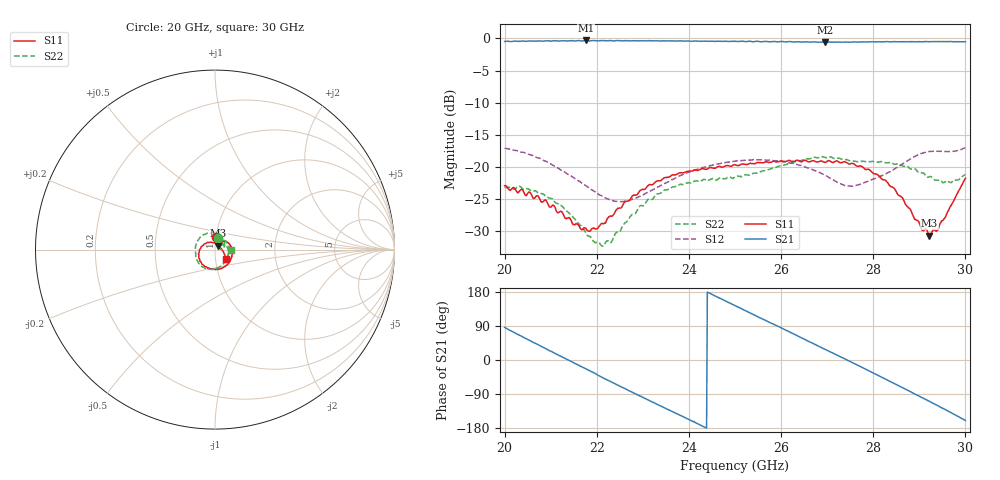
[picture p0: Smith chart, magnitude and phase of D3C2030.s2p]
! 4/13/2021 3:11:42 PM
! C:\USERS\DITOM\DESKTOP\SINGLE JUNCTION ISOLATOR DATA\20.0 - 30.0 GHZ (D3I2030).S2P
! CHANNEL.1
! TR.MEASUREMENT
! CORRECTED.DATA
# GHZ S RI R 50.0
! FREQ.GHZ  S11RE  S11IM  S21RE  S21IM  S12RE  S12IM  S22RE  S22IM
!; PortSelection: Port_12
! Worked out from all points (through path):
!   601 points, 20 GHz to 30 GHz, reference 50 ohm
!   highest |S21| = -0.31 dB at 21.77 GHz (marker M1); lowest = -0.6 dB at 26.95 GHz (marker M2)
!   lowest |S11| = -30.8 dB at 29.22 GHz (marker M3), VSWR 1.06, Z = 51.9 + j2.3 ohm
!   |S11| at or under -10 dB: start of sweep to end of sweep
!   |S22| runs from -32.4 to -18.4 dB; largest |S21 - S12| = 1.1
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20  0.00492 0.0708  0.0663 0.9457  0.0745 -0.1178  0.0187 0.0667
20.4  0.0236 0.0606  0.4715 0.8298  -0.00185 -0.1294  0.0425 0.0516
20.91667  0.0367 0.0385  0.8435 0.4574  -0.0806 -0.0739  0.0532 0.0236
21.28333  0.0328 0.0258  0.9555 0.0958  -0.0913 -0.0122  0.0468 0.0082
21.66667  0.0248 0.0207  0.9123 -0.2894  -0.0629 0.0404  0.0345 0.00198
21.76667  0.0239 0.0227  0.8854 -0.3844  -0.0512 0.0491  0.03 0.00248
22.13333  0.0192 0.0304  0.6569 -0.7039  -0.00124 0.0584  0.0222 0.00898
22.6  0.0296 0.0435  0.2519 -0.9281  0.0482 0.0237  0.0273 0.0235
23.35  0.0642 0.0436  -0.4678 -0.8335  0.0239 -0.0658  0.0564 0.0246
24.18333  0.0933 0.00397  -0.9322 -0.1985  -0.083 -0.0464  0.0764 -0.0123
24.6  0.0961 -0.0227  -0.9281 0.2079  -0.104 0.00981  0.0707 -0.0346
25  0.0924 -0.0469  -0.7648 0.5647  -0.0876 0.0668  0.0636 -0.0535
25.46667  0.0763 -0.0748  -0.419 0.8541  -0.0319 0.1084  0.0506 -0.0732
25.83333  0.0573 -0.0946  -0.0747 0.9457  0.0218 0.1092  0.0331 -0.092
26.2  0.0318 -0.1065  0.2765 0.9048  0.0655 0.0841  0.00425 -0.1069
26.66667  -0.0105 -0.1104  0.66 0.6664  0.0893 0.0337  -0.0487 -0.1063
26.95  -0.0337 -0.1025  0.8214 0.4442  0.0857 0.00624  -0.0783 -0.0884
27.61667  -0.0843 -0.0582  0.9214 -0.1825  0.068 -0.0209  -0.1086 -0.0183
28.35  -0.0677 0.0224  0.5296 -0.778  0.065 -0.0634  -0.0865 0.0642
28.8  -0.0207 0.0417  0.1134 -0.9377  0.0415 -0.1067  -0.0307 0.0913
29.21667  0.0187 0.0222  -0.3047 -0.8928  -0.0226 -0.1294  0.0255 0.0794
30  0.0609 -0.0535  -0.883 -0.33  -0.1134 -0.0832  0.0868 0.000277
